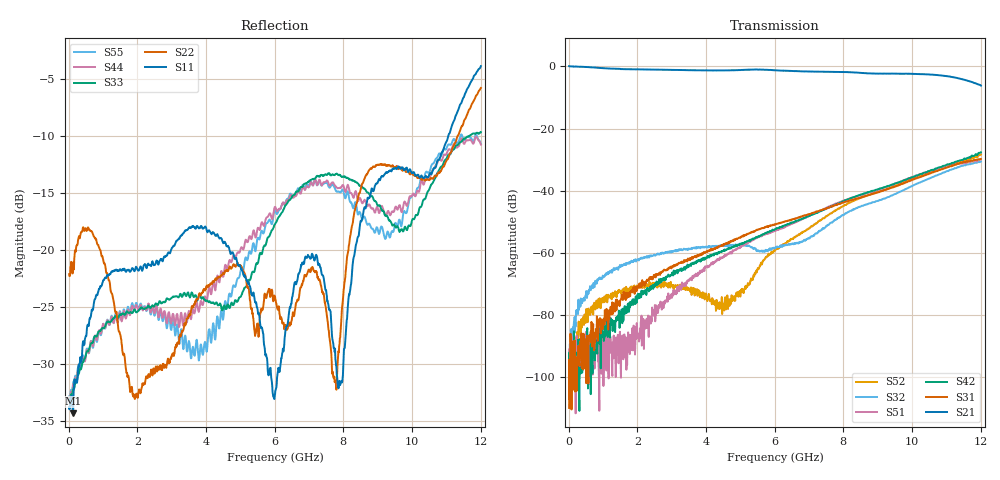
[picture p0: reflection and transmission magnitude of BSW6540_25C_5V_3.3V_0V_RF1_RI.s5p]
! Agilent Technologies	N5230C	MY49001333	A.09.33.09
!	Test time	=	2026-05-06 10:00
!	Product	=	BSW6540
!	Temp	=	25C
!	VDD	=	5
!	Control_High	=	3.3
!	Control_Low	=	0
!	Logic	=	RF1
!	Port1	=	RFC
!	Port2	=	RF1
!	Port3	=	RF2
!	Port4	=	RF3
!	Port5	=	RF4
!	V1	=	3.3 / 0
!	V2	=	3.3 / 0
!S5P File: Measurements: <S11,S12,S13,S14,S15>,
!<S21,S22,S23,S24,S25>,
!<S31,S32,S33,S34,S35>,
!<S41,S42,S43,S44,S45>,
!<S51,S52,S53,S54,S55>;
# HZ S RI R 50
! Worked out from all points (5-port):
!   1201 points, 10 MHz to 12.01 GHz, reference 50 ohm
!   strongest paths, dB at 10 MHz, 3.01 GHz, 6.01 GHz, 9.01 GHz, 12.01 GHz:
!     S21: 0.1, -1.1, -1.3, -2.3, -6.2
!     S31: -109.9, -64.7, -50.9, -40.5, -29.8
!     S42: -97.4, -66.4, -52.5, -39.6, -27.7
!     S51: -91.1, -74.2, -52.9, -39.8, -29.9
!     S32: -94.5, -59.7, -58.6, -43.3, -30.6
!     S52: -95.4, -70.5, -59.2, -40.5, -28.4
!   lowest |S11| = -34.3 dB at 120 MHz (marker M1), VSWR 1.04, Z = 51.8 - j0.845 ohm
!   |S11| at or under -10 dB: start of sweep to 11.06 GHz
